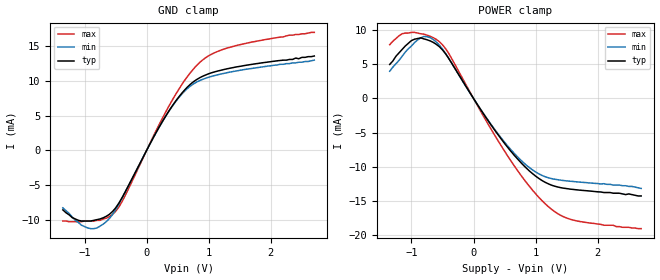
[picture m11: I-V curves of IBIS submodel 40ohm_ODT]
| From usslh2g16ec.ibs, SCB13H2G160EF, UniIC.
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| SUBMODEL 40ohm_ODT
[Submodel]   40ohm_ODT
Submodel_type  Dynamic_clamp
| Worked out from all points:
|   GND clamp passes 1 mA (typ) near -0.06 V on its own axis
|   POWER clamp passes 1 mA (typ) near -0.07 V on its own axis
[GND Clamp]
|Voltage   I(typ)   I(min)   I(max)
-1.35V    -8.6mA     -8.3mA     -10.2mA
-1.2V     -9.7mA     -9.6mA     -10.3mA
-950mV    -10.2mA    -11.2mA    -10.2mA
-800mV    -10mA      -11.2mA    -10.1mA
-650mV    -9.52mA    -10.29mA   -9.79mA
-400mV    -6.89mA    -6.98mA    -7.46mA
100mV     1.707mA    1.705mA    1.885mA
400mV     6.238mA    6.182mA    7.036mA
650mV     9.06mA     8.86mA     10.56mA
950mV     10.86mA    10.39mA    13.35mA
1.45V     12.03mA    11.45mA    15.12mA
2.7V      13.6mA     13mA       17mA
[POWER Clamp]
|Voltage   I(typ)   I(min)   I(max)
-1.35V    5mA        4mA        7.9mA
-1.15V    7.2mA      6.2mA      9.5mA
-1V       8.5mA      7.7mA      9.7mA
-850mV    8.9mA      8.9mA      9.5mA
-700mV    8.46mA     8.93mA     9.14mA
-400mV    5.886mA    5.893mA    6.62mA
150mV     -2.112mA   -2.075mA   -2.431mA
550mV     -7.172mA   -6.963mA   -8.44mA
900mV     -10.64mA   -10.14mA   -12.89mA
1.2V      -12.5mA    -11.62mA   -15.83mA
1.65V     -13.39mA   -12.22mA   -17.94mA
2.7V      -14.3mA    -13.2mA    -19.1mA
